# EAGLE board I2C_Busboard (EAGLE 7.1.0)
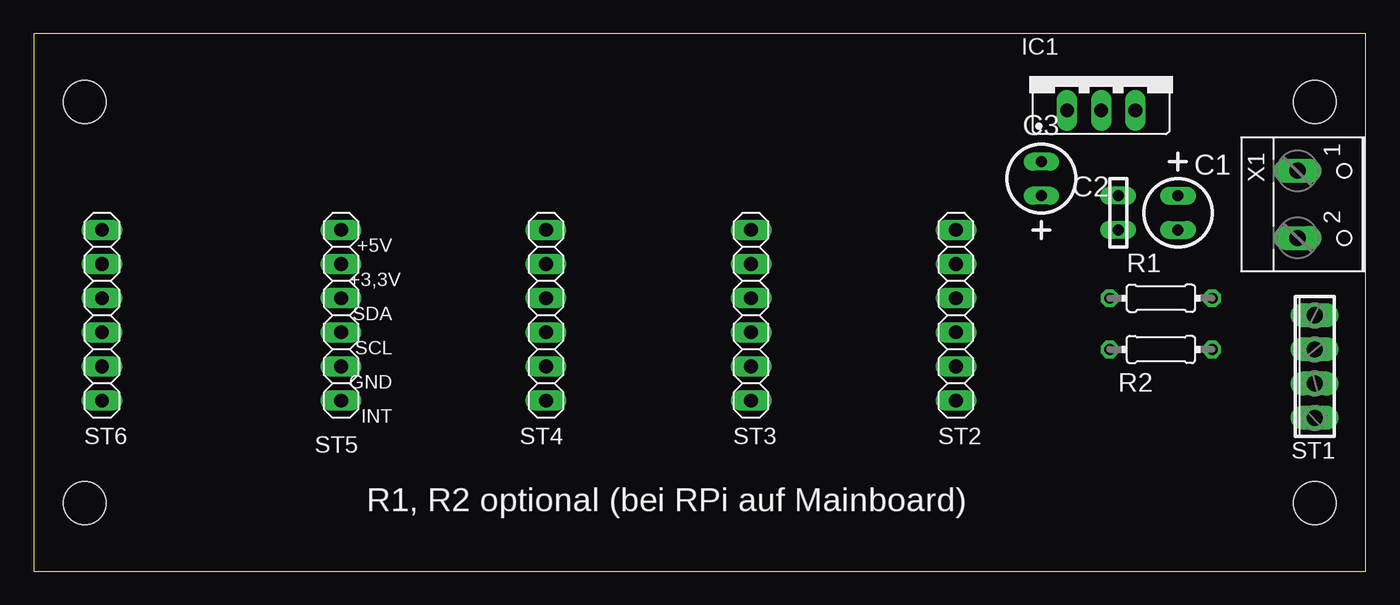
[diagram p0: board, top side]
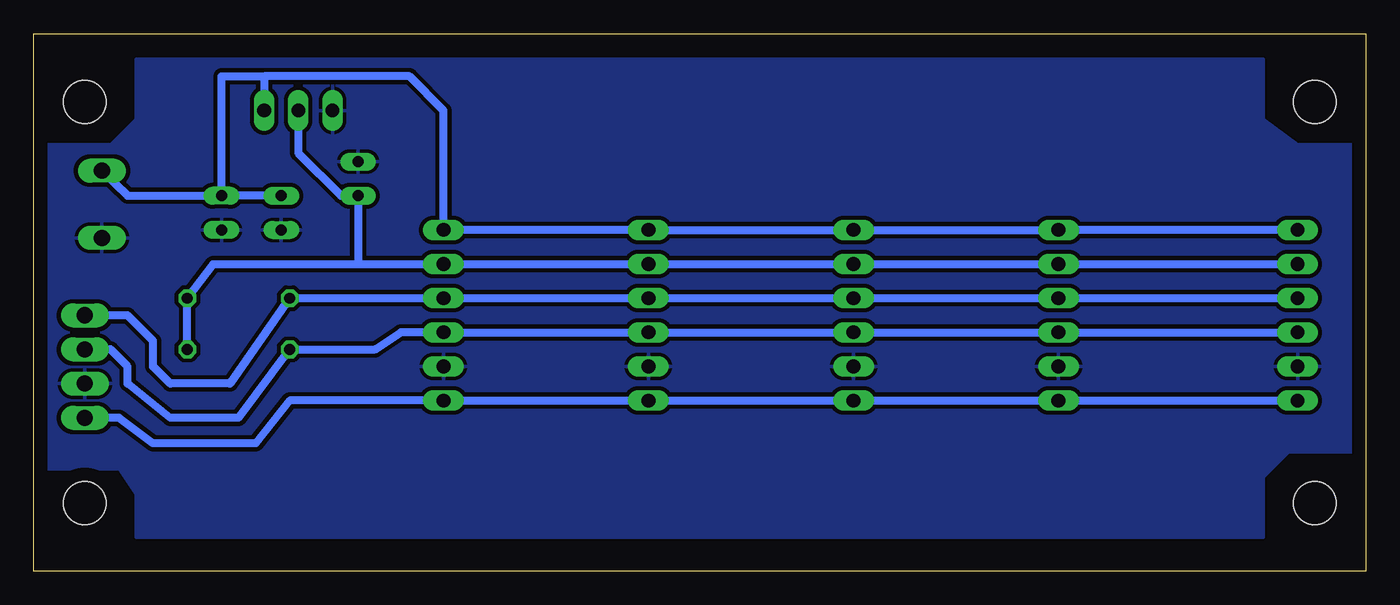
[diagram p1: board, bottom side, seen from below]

Size 99.06 x 40.01 mm. Coordinates in mm from the lower left corner, seen from the top.
Outline: 99.06,0 99.06,40.01 0,40.01 0,0 99.06,0
Copper layers (1*16): Top 0.035mm / dielectric 1.5mm / Bottom 0.035mm
Design rules "default": minimum track width 10mil, minimum drill 24mil, track to track 12mil, track to pad 12mil, pad to pad 12mil, via to via 12mil, smd to smd 8mil, copper to edge 40mil, drill to drill 8mil, minimum pad ring 10mil, minimum via ring 8mil, stop-mask expansion 4mil, vias tented up to drill 0mil, thermal gap 10mil
Holes 3.17 mm at 95.25,5.08 95.25,34.92 3.81,5.08 3.81,34.92

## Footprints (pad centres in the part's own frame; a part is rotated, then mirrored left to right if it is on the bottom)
E2,5 = drill 0.813 pad 1.27 long: N 2.54,0; P 0,0
C2,5 = drill 0.813 pad 1.27 long: 1 2.54,0; 2 0,0
78XXS = drill 1.016 long: GND 0,-2.54; IN -2.54,-2.54; OUT 2.54,-2.54
0204/7 = drill 0.813 octagon: 1 -3.81,0; 2 3.81,0
4POL254 = drill 1.2 long: 1 -3.81,0; 2 -1.27,0; 3 1.27,0; 4 3.81,0
1X06L = drill 1.016 long: 1 -6.35,0; 2 -3.81,0; 3 -1.27,0; 4 1.27,0; 5 3.81,0; 6 6.35,0
W237-102 = drill 1.194 long: 1 -2.5,-1.27; 2 2.5,-1.27

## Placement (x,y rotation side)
C1  100µ  [E2,5]  85.09,27.94 270 top
C2  100n  [C2,5]  80.64,27.94 270 top
C3  47µ  [E2,5]  74.93,27.94 90 top
IC1  LD1117V33  [78XXS]  79.38,36.83 0 top
R1  4,7k  [0204/7]  83.82,20.32 0 top
R2  4,7k  [0204/7]  83.82,16.51 0 top
ST1  [4POL254]  95.25,15.24 90 top
ST2  [1X06L]  68.58,19.05 270 top
ST3  [1X06L]  53.34,19.05 270 top
ST4  [1X06L]  38.1,19.05 270 top
ST5  [1X06L]  22.86,19.05 270 top
ST6  [1X06L]  5.08,19.05 270 top
X1  [W237-102]  95.25,27.3 270 top

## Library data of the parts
C1-C3 ST2-ST6 = mc-parts
IC1 = v-reg
R1 R2 = rcl
ST1 = con-phoenix-254
X1 = con-wago-500

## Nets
GND: C1.N C2.1 C3.N IC1.IN ST1.2 ST2.5 ST3.5 ST4.5 ST5.5 ST6.5 X1.2
INT: ST1.1 ST2.6 ST3.6 ST4.6 ST5.6 ST6.6
SCL: R2.1 ST1.3 ST2.4 ST3.4 ST4.4 ST5.4 ST6.4
SDA: R1.1 ST1.4 ST2.3 ST3.3 ST4.3 ST5.3 ST6.3
VCC: C3.P IC1.GND R1.2 R2.2 ST2.2 ST3.2 ST4.2 ST5.2 ST6.2
VCC1: C1.P C2.2 IC1.OUT ST2.1 ST3.1 ST4.1 ST5.1 ST6.1 X1.1

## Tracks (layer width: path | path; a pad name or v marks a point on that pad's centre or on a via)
GND
  pour Bottom: 7.62,2.54 91.44,2.54 91.44,5.71 92.71,7.62 99.06,7.62 99.06,31.75 93.34,31.75 91.44,33.66 91.44,38.1 7.62,38.1 7.62,33.66 5.08,31.75 0.64,31.75 0.64,8.89 5.71,8.89 7.62,6.99
INT
  Bottom 0.61: ST6.6 ST5.6 ST4.6 ST3.6 ST2.6 80.01,12.7 82.55,9.53 90.17,9.53 92.71,11.43 ST1.1
SCL
  Bottom 0.61: ST6.4 ST5.4 ST4.4 ST3.4 ST2.4 71.75,17.78 73.66,16.51 R2.1 83.82,11.43 88.9,11.43 92.08,13.97 92.08,15.24 93.34,16.51 ST1.3
SDA
  Bottom 0.61: ST6.3 ST5.3 ST4.3 ST3.3 ST2.3 R1.1 84.45,13.97 88.9,13.97 90.17,15.24 90.17,17.14 92.08,19.05 ST1.4
VCC
  Bottom 0.61: ST6.2 15.24,22.86 ST5.2 ST4.2 ST3.2 ST2.2 74.93,22.86 | R2.2 R1.2 85.72,22.86 74.93,22.86 | 74.93,22.86 C3.P 76.2,27.94 79.38,31.11 IC1.GND
VCC1
  Bottom 0.61: ST6.1 10.16,25.4 ST5.1 ST4.1 ST3.1 ST2.1 68.58,34.29 71.12,36.83 81.92,36.83 | C2.2 C1.P | C1.P 92.08,27.94 X1.1 | C1.P 85.09,36.83 81.92,36.83 | 81.92,36.83 IC1.OUT

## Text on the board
tPlace: +5V | +3,3V | SDA | SCL | GND | INT | R1, R2 optional (bei RPi auf Mainboard)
